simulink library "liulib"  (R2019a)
settings: Solver=ode45  StartTime=0.0  StopTime=10.0  RelTol=1e-3  EnableMultiTasking=on
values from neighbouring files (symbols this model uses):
  ag = NaN(L.ng,1)    [bdet.m]
  D = meqp()    [fbtp.m]
  dr2FA = dr2Fs(1:nA,1)    [asxycs.m]
  drzFA = drzFs(1:nA,1)    [asxycs.m]
  dz = dzxs(is)    [asxycsJac.m]    (also in bintc.m = (z - zx(kz))/dzx)
  dz2FA = dz2Fs(1:nA,1)    [asxycs.m]
  err = [IaeH            ; IoeH               ; IueH               ; DeH               ; FeH            ; BeH               ; BeH               ; BeH               ; CeH               ; CeH               ; CeH               ; VeH                ; VeH                ; VeH               ]    [fbtopt.m]
  FA = Fs(1:nA,1)    [asxycs.m]    (also in bfhelp.m = [-1                        0        0       ])
  FB = [0                         1        1       ]    [bfhelp.m]
  Fx = meqFx(L,Iy,[Ia;Iu])    [bdet.m]    (also in bfhelp.m = zeros(n+2,3); Fx(2:end-1,2) = FN)
  FX = Fs(nA+1:ns,1)    [asxycs.m]
  IpD = LXs.Ip    [fbtinit.m]
  Iy = LXt.Iy    [bdet.m]    (also in fbtinit.m = meqinitIy(L,LXs.t,IpD,bbs,LXs.capaj))
  L = fbtc(P,G)    [fbt.m]    (also in fbtc.m = meqc(P,G); fbte.m = varargout{1})
  nA = numel(rA)    [asxycs.m]
  niter = L.P.itercs    [asxycs.m]
  Opy = logical(Opy)    [bfct.m]    (also in bfdoublet.m = Opy==1 | Opy==2)
  rA = rs(1:nA,1)    [asxycs.m]    (also in fbtptcv.m = (rA1 + 3*rA2)/4)
  rX = rs(nA+1:ns,1)    [asxycs.m]    (also in fbtptcv.m = rzbro(iX,1); fbtxana.m = r0)
  zA = zs(1:nA,1)    [asxycs.m]    (also in fbtptcv.m = (zA1 + 3*zA2)/4)
  zX = zs(nA+1:ns,1)    [asxycs.m]    (also in fbtptcv.m = rzbro(iX,2); fbtxana.m = 0)
undefined symbols (not defined in the file or in its folder): aminor, aq, aW, Bm, bp, bpli2, Brn, Brrn, Brzn, bt, Bzn, Bzrn, Bzzn, delta, deltal, deltau, dzg, epsilon, Ff, Fn, Ft, Ft0, FW, Ie, Ip, iqQ, iTQ, jtorQ, kappa, lB, li, lp, lX, mu, nX, PpQ, PQ, Q0Q, Q1Q, Q2Q, Q3Q, Q4Q, q95, qmin, raQ, raqmin, rB, rbary, rBt, repmat, rgeom, rIp, rIpD, Row, rq, rS, rst, rYD, TQ, TTpQ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
libraries: $bdroot x53, mkllib x48, simulink x7
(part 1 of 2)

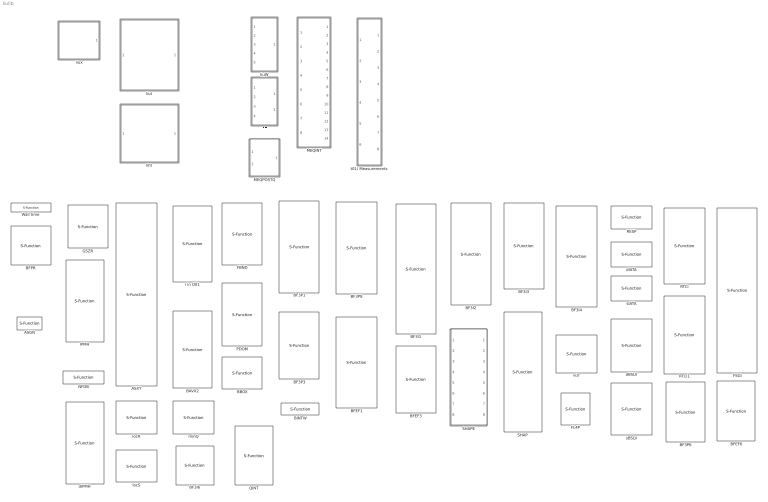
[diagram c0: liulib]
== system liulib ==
  ASGN : S-Function  FunctionName=sasgncsf  Parameters=iu  SFunctionDeploymentMode=off  EnableBusSupport=off  mask{iu=0}
  ASXY : S-Function  FunctionName=sasxycsf  Parameters=rx zx dr dz idr idz Oasx daxm  SFunctionDeploymentMode=off  EnableBusSupport=off  mask{rx=L.G.rx, zx=L.G.zx, dr=L.drx, dz=L.dzx, idr=L.idrx, idz=L.idzx, Oasx=L.Oasx, daxm=L.P.daxm}
      mask prompts: rx "rx [28]"; zx "zx [65]"
      mask help: Axis and Saddle point finder on xy grid
  BAVX2 : S-Function  FunctionName=sbavx2csf  Parameters=a  SFunctionDeploymentMode=off  EnableBusSupport=off  mask{a=0}
      mask prompts: a "alpha"
  BBOX : S-Function  FunctionName=sbboxcsf  Parameters=z r  SFunctionDeploymentMode=off  EnableBusSupport=off  mask{z=L.zy, r=L.ry}
  BF3I1 : S-Function  FunctionName=sbf3i1csf  Parameters=r ir nz nr  SFunctionDeploymentMode=off  EnableBusSupport=off  mask{r=L.ry, ir=L.iry, nz=L.nzy, nr=L.nry}
      mask prompts: r "r inner grid"; ir "ir inner grid"; nz "nzy"; nr "nry"
  BF3I2 : S-Function  FunctionName=sbf3i2csf  SFunctionDeploymentMode=off  EnableBusSupport=off
  BF3I3 : S-Function  FunctionName=sbf3i3csf  Parameters=idsx  SFunctionDeploymentMode=off  EnableBusSupport=off  mask{idsx=L.idsx}
  BF3I4 : S-Function  FunctionName=sbf3i4csf  Parameters=nzy nry  SFunctionDeploymentMode=off  EnableBusSupport=off  mask{nzy=L.nzy, nry=L.nry}
  BF3I6 : S-Function  FunctionName=sbf3i6csf  SFunctionDeploymentMode=off  EnableBusSupport=off
  BF3P1 : S-Function  FunctionName=sbf3p1csf  Parameters=ry iry nzy nry  SFunctionDeploymentMode=off  EnableBusSupport=off  mask{ry=L.ry, iry=L.iry, nzy=L.nzy, nry=L.nry}
      mask prompts: ry "ry inner grid"; iry "iry inner grid"
  BF3P3 : S-Function  FunctionName=sbf3p3csf  Parameters=idsx  SFunctionDeploymentMode=off  EnableBusSupport=off  mask{idsx=L.idsx}
  BF3P6 : S-Function  FunctionName=sbf3p6csf  SFunctionDeploymentMode=off  EnableBusSupport=off
  BF3P8 : S-Function  FunctionName=sbf3p8csf  Parameters=ids iry  SFunctionDeploymentMode=off  EnableBusSupport=off  mask{ids=L.idsx, iry=L.iry}
      mask prompts: ids "r inner grid"; iry "ir inner grid"
  BFEF1 : S-Function  FunctionName=sbfef1csf  Parameters=ry iry nzy nry nP nT  SFunctionDeploymentMode=off  EnableBusSupport=off  mask{ry=L.ry, iry=L.iry, nzy=L.nzy, nry=L.nry, nP=L.P.bfp(1), nT=L.P.bfp(2)}
      mask prompts: ry "ry inner grid"; iry "iry inner grid"
  BFEF3 : S-Function  FunctionName=sbfef3csf  Parameters=ids nP nT  SFunctionDeploymentMode=off  EnableBusSupport=off  mask{ids=L.idsx, nP=L.P.bfp(1), nT=L.P.bfp(2)}
  BFEF6 : S-Function  FunctionName=sbfef6csf  Parameters=nP nT nq  SFunctionDeploymentMode=off  EnableBusSupport=off  mask{nP=L.P.bfp(1), nT=L.P.bfp(2), nq=L.nq}
  BFPR : S-Function  FunctionName=sbfprcsf  SFunctionDeploymentMode=off  EnableBusSupport=off
  BINTW : S-Function  FunctionName=sbintcsf  Parameters=kxW cWx nzx  SFunctionDeploymentMode=off  EnableBusSupport=off  mask{kxW=L.kxW, cWx=L.cWx, nzx=L.nzx}
  FBND : S-Function  FunctionName=sfbndcsf  Parameters=rl zl  SFunctionDeploymentMode=off  EnableBusSupport=off  mask{rl=L.G.rl, zl=L.G.zl}
  FE : Subsystem  Variant=on
  FL4P : S-Function  FunctionName=sfl4pcsf  Parameters=kl cl nz  SFunctionDeploymentMode=off  EnableBusSupport=off  mask{kl=int32(L.kxl-1), cl=L.clx, nz=L.nzx}
      mask prompts: kl "kl 0-based"; cl "cl [4][]"
  FSGI : S-Function  FunctionName=sfsgicsf  Parameters=idoq  SFunctionDeploymentMode=off  EnableBusSupport=off  mask{idoq=1/L.doq}
      mask help: Flux Surface Geometric Integrals
  GSZR : S-Function  FunctionName=sgszrcsf  Parameters=cx cq cr cs ci co  SFunctionDeploymentMode=off  EnableBusSupport=off  mask{cx=L.cx, cq=L.cq, cr=L.cr, cs=L.cs, ci=L.ci, co=L.co}
      mask help: Grad-Shafranov equation on RZ grid
  IPMH : S-Function  FunctionName=sipmhcsf  Parameters=Ahd Aed Ahe Aeh Ahh uAhh nit  SFunctionDeploymentMode=off  EnableBusSupport=off  mask{Ahd=L.Ahd, Aed=L.Aed, Ahe=L.Ahe, Aeh=L.Aeh, Ahh=L.Ahh, uAhh=L.uAhh, nit=L.P.iterh}
      mask prompts: nit "Maximum iteration #"
  MEQINT : Subsystem
  MEQPOSTQ : Subsystem  TreatAsAtomicUnit=on  VariantControl=liuITERQMODEvariant1
  NFDB : S-Function  FunctionName=snfdbcsf  Parameters=nz nr  SFunctionDeploymentMode=off  EnableBusSupport=off  mask{nz=L.nzx, nr=L.nrx}
  PDOM : S-Function  FunctionName=spdomcsf  SFunctionDeploymentMode=off  EnableBusSupport=off
      mask help: Plasma DOmain finder
  QINT : S-Function  FunctionName=sqintcsf  Parameters=rx zx inM  SFunctionDeploymentMode=off  EnableBusSupport=off  mask{rx=L.rx, zx=L.zx, inM=L.inM}
  RESP : S-Function  FunctionName=srespcsf  Parameters=A B nr ng  SFunctionDeploymentMode=off  EnableBusSupport=off  mask{A=L.Wr.*L.Mry, B=L.P.fdz*(L.Wr.*L.Mdzry), nr=L.nr, ng=L.ng}
      mask prompts: A "Mry"; B "Mdzry"
  RTCI : S-Function  FunctionName=srtcicsf  Parameters=c s da nr nz  SFunctionDeploymentMode=off  EnableBusSupport=off  mask{c=L.cdrq, s=L.cdzq, da=L.drx, nr=L.nrx, nz=L.nzx}
      mask prompts: c "cos(theta)*dr"; s "sin(theta)*dz"; da "delta a max"
      mask help: Real-Time Contour Integration
  RTCI1 : S-Function  FunctionName=srtci1csf  SFunctionDeploymentMode=off  EnableBusSupport=off
  SHAP : S-Function  FunctionName=sshapcsf  Parameters=npq noq  SFunctionDeploymentMode=off  EnableBusSupport=off  mask(Computes shape parameters from rq,zq contours){npq=L.npq, noq=L.noq}
      mask help: See shapmex.c, shap.c
  SHAPE : Subsystem  mask(meqshape){npq=L.npq, noq=L.noq}
      mask help: Calculates LCFS shape information. See meqshape.m for details
  Wall time : S-Function  FunctionName=swclkcsf  Parameters=f  SFunctionDeploymentMode=off  EnableBusSupport=off  mask{f=1e6}
      mask prompts: f "Factor (e.g. 1000 for ms)"
  dBSLV : S-Function  FunctionName=dbslvcsf  Parameters=niter  SFunctionDeploymentMode=off  EnableBusSupport=off  mask{niter=L.P.iters}
  dIATA : S-Function  FunctionName=diatacsf  SFunctionDeploymentMode=off  EnableBusSupport=off
  dIPMH : S-Function  FunctionName=dipmhcsf  Parameters=Ahd Aed Ahe Aeh Ahh uAhh nit  SFunctionDeploymentMode=off  EnableBusSupport=off  mask{Ahd=0, Aed=0, Ahe=0, Aeh=0, Ahh=0, uAhh=0, nit=0}
      mask prompts: nit "Maximum iteration #"
  l in OX1 : S-Function  FunctionName=sbavxcsf  Parameters=a  SFunctionDeploymentMode=off  EnableBusSupport=off  mask{a=0}
      mask prompts: a "alpha"
  liht : Subsystem  TreatAsAtomicUnit=on
  liuW : Subsystem  TreatAsAtomicUnit=on
  liut : Subsystem  TreatAsAtomicUnit=on
  liux : Subsystem
  locR : S-Function  FunctionName=slocRcsf  Parameters=nR naR  SFunctionDeploymentMode=off  EnableBusSupport=off  mask{nR=numel(L.P.iqR), naR=1}
  locS : S-Function  FunctionName=slocScsf  SFunctionDeploymentMode=off  EnableBusSupport=off
  minQ : S-Function  FunctionName=sminQcsf  Parameters=nmin  SFunctionDeploymentMode=off  EnableBusSupport=off  mask{nmin=1}
  sBSLV : S-Function  FunctionName=sbslvcsf  Parameters=niter  SFunctionDeploymentMode=off  EnableBusSupport=off  mask{niter=L.P.iters}
  sIATA : S-Function  FunctionName=siatacsf  SFunctionDeploymentMode=off  EnableBusSupport=off
  t01/ Measurements : Subsystem
  vizr : S-Function  FunctionName=svizrcsf  Parameters=ry iry dr dz nr nz  SFunctionDeploymentMode=off  EnableBusSupport=off  mask{ry=L.ry, iry=L.iry, dr=L.drx, dz=L.dzx, nr=L.nrx, nz=L.nzx}
      mask prompts: ry "r inner grid"; iry "ir inner grid"

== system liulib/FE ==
  Yd : Inport
  Ie : Inport  Port=2
  Ip : Inport  Port=3
  sIp : Inport  Port=4
  FE ipm : Subsystem  VariantControl=liuHFCTMODEvariant2
  FE ipm double : Subsystem  VariantControl=liuHFCTMODEvariant3
  FE lsq : Subsystem  VariantControl=liuHFCTMODEvariant1
  Jh : Outport
  Je : Outport  Port=2

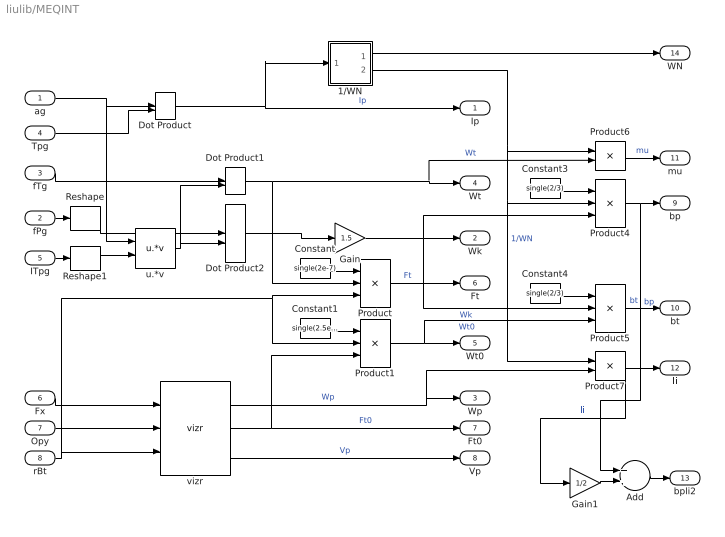
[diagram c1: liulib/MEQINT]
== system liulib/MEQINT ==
  ag : Inport
  fPg : Inport  Port=2
  fTg : Inport  Port=3
  Tpg : Inport  Port=4
  ITpg : Inport  Port=5
  Fx : Inport  Port=6
  Opy : Inport  Port=7
  rBt : Inport  Port=8
  1/WN : Subsystem
  Add : Sum
  Constant : Constant  Value=single(2e-7)  OutDataTypeStr=single
  Constant1 : Constant  Value=single(2.5e6)  OutDataTypeStr=single
  Constant3 : Constant  Value=single(2/3)  OutDataTypeStr=single
  Constant4 : Constant  Value=single(2/3)  OutDataTypeStr=single
  Dot Product : DotProduct
  Dot Product1 : DotProduct
  Dot Product2 : DotProduct
  Gain : Gain  Gain=1.5
  Gain1 : Gain  Gain=1/2
  Product : Product  Inputs=**/
  Product1 : Product  Inputs=3
  Product4 : Product  Inputs=3
  Product5 : Product  Inputs=**/
  Product6 : Product
  Product7 : Product
  Reshape : Reshape
  Reshape1 : Reshape
  u.*v : mkllib/u.*v
  vizr : $bdroot/vizr  ry=L.ry  iry=L.iry  dr=L.drx  dz=L.dzx  nr=L.nrx  nz=L.nzx
  Ip : Outport
  Wk : Outport  Port=2
  Wp : Outport  Port=3
  Wt : Outport  Port=4
  Wt0 : Outport  Port=5
  Ft : Outport  Port=6
  Ft0 : Outport  Port=7
  Vp : Outport  Port=8
  bp : Outport  Port=9
  bt : Outport  Port=10
  mu : Outport  Port=11
  li : Outport  Port=12
  bpli2 : Outport  Port=13
  WN : Outport  Port=14
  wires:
  1/WN/1(WN) -> WN/1
  Gain1/1 -> Add/2
  Add/1 -> bpli2/1
  vizr/3 -> Vp/1  "Vp"
  Fx/1 -> vizr/1
  rBt/1 -> Product1/2, Product/3, vizr/3
  ag/1 -> u.*v/1, Dot Product/1
  Tpg/1 -> Dot Product/2
  u.*v/1 -> Dot Product1/2, Dot Product2/2
  Dot Product/1 -> 1/WN/1(Ip), Ip/1  "Ip"
  Dot Product2/1 -> Gain/1
  vizr/1 -> Product7/2, Wp/1  "Wp"
  Dot Product1/1 -> Product/2, Product6/2, Wt/1  "Wt"
  fTg/1 -> Dot Product1/1
  vizr/2 -> Ft0/1, Product1/3  "Ft0"
  Constant/1 -> Product/1
  Product/1 -> Ft/1  "Ft"
  Constant1/1 -> Product1/1
  Product1/1 -> Product5/3, Wt0/1  "Wt0"
  Constant3/1 -> Product4/1
  Product4/1 -> bp/1, Add/1  "bp"
  Product5/1 -> bt/1  "bt"
  Constant4/1 -> Product5/1
  Product6/1 -> mu/1  "mu"
  Product7/1 -> li/1, Gain1/1  "li"
  Gain/1 -> Product5/2, Product4/3, Wk/1  "Wk"
  1/WN/2(1/WN) -> Product6/1, Product7/1, Product4/2  "1/WN"
  fPg/1 -> Reshape/1
  ITpg/1 -> Reshape1/1
  Reshape/1 -> Dot Product2/1
  Reshape1/1 -> u.*v/2
  Opy/1 -> vizr/2

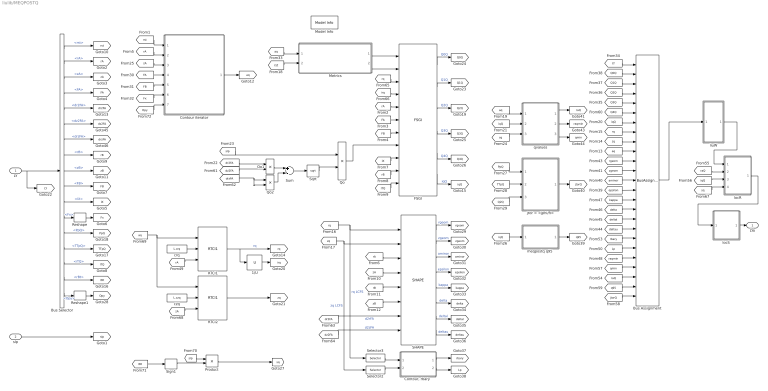
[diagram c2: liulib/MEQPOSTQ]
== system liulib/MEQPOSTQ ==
  LY : Inport
  sIp : Inport  Port=2
  1/U : mkllib/1//U
  Bus Assignment : BusAssignment  AssignedSignals=Q0Q,Q1Q,Q2Q,Q3Q,Q4Q,iqQ,rq,zq,aq,rgeom,zgeom,aminor,epsilon,kappa,delta,deltal,deltau,rbary,lp,raqmin,qmin,raQ,q95,jtorQ
  Bus Selector : BusSelector  OutputSignals=rst,rA,zA,FA,dr2FA,dz2FA,drzFA,rB,zB,FB,lX,Fx,PpQ,TTpQ,iTQ,rBt,Opy
  Contour iterator : Subsystem
  "Contour, rbary " : Subsystem
  FSGI : $bdroot/FSGI  idoq=1/L.doq
  Metrics : Subsystem
  Model Info : simulink/Model-Wide Utilities/Model Info  Frame=on  DisplayStringWithTags=|  HorizontalTextAlignment=Center  LeftAlignmentValue=0.5
      | Model Info
      | %<Creator>
      | %<ModifiedBy>
      | %<ModifiedDate>
      | %<ModifiedComment>
      | %<ModelVersion>
  Product : Product
  Qo : Product  Inputs=**
  Qo1 : Product  Inputs=**
  Qo2 : Product  Inputs=**
  RTCI1 : $bdroot/RTCI1  SFunctionModules=''
  RTCI2 : $bdroot/RTCI1  SFunctionModules=''
  Reshape : Reshape  OutputDimensions=L.nzx*L.nrx
  Reshape1 : Reshape  OutputDimensions=L.nzy*L.nry
  SHAPE : $bdroot/SHAPE  npq=L.npq  noq=L.noq
  Selector2 : Selector  NumberOfDimensions=2  InputPortWidth=3  IndexOptions=Select all,Index vector (dialog)  Indices=[1 3],L.npq  OutputSizes=1,1
  Selector3 : Selector  NumberOfDimensions=2  InputPortWidth=3  IndexOptions=Select all,Index vector (dialog)  Indices=[1 3],L.npq  OutputSizes=1,1
  Sign1 : Signum
  Sqrt : Sqrt
  Sum : Sum  Inputs=+-
  crq : Constant  Value=L.crq  OutDataTypeStr=single
  czq : Constant  Value=L.czq  OutDataTypeStr=single
  jtor = <jphi/R> : Subsystem
  liuW : Subsystem  Variant=on  VariantControl=Variant1
  locR : Subsystem  Variant=on  VariantControl=Variant1
  locS : Subsystem  Variant=on  VariantControl=Variant1
  "meqpostq q95 " : Subsystem
  qvalues : Subsystem
  LYo : Outport
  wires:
  "Contour, rbary "/1(rbary) -> [rbary]
  "Contour, rbary "/2(Lp) -> [Lp]
  qvalues/2(raqmin) -> [raqmin]
  qvalues/3(qmin) -> [qmin]
  [iTQ] -> FSGI/11
  FSGI/1 -> [Q0Q]  "Q0Q"
  Bus Selector/5 -> [dr2FA]  "<dr2FA>"
  SHAPE/3 -> [aminor]  "aminor"
  Bus Selector/4 -> [FA]  "<FA>"
  SHAPE/1 -> [rgeom]  "rgeom"
  SHAPE/8 -> [deltau]  "deltau"
  [rq] -> SHAPE/1, Selector3/1  "rq LCFS"
  [sIp] -> Qo/1
  [iqQ] -> qvalues/2(iqQ)
  Selector2/1 -> "Contour, rbary "/2(zq)
  Bus Selector/2 -> [rA]  "<rA>"
  SHAPE/6 -> [delta]  "delta"
  [rB] -> FSGI/10
  Bus Selector/3 -> [zA]  "<zA>"
  FSGI/4 -> [Q3Q]  "Q3Q"
  Sum/1 -> Sqrt/1
  [zq] -> SHAPE/2, Selector2/1  "zq LCFS"
  [FB] -> FSGI/7
  Metrics/1(da^2/pdp = M1q) -> FSGI/1
  FSGI/6 -> [iqQ]  "iqQ"
  Sqrt/1 -> Qo/2
  [dz2FA] -> SHAPE/8  "d2zFA"
  [sq] -> qvalues/3(sq)
  [aq] -> qvalues/1(aq)
  [dr2FA] -> Qo1/1
  [rst] -> Metrics/2(rst)
  [rB] -> SHAPE/5
  FSGI/2 -> [Q1Q]  "Q1Q"
  [zA] -> SHAPE/4
  Qo1/1 -> Sum/1
  Selector3/1 -> "Contour, rbary "/1(rq)
  SHAPE/4 -> [epsilon]  "epsilon"
  SHAPE/2 -> [zgeom]  "zgeom"
  SHAPE/7 -> [deltal]  "deltal"
  [drzFA] -> Qo2/2, Qo2/1
  [rA] -> SHAPE/3
  [rA] -> FSGI/5
  Qo/1 -> FSGI/8
  [FA] -> FSGI/6
  Qo2/1 -> Sum/2
  Metrics/2(((da^2/2do)^2+a^2)/(da^2/pdp) = M2q) -> FSGI/2
  [zB] -> SHAPE/6
  [lX] -> FSGI/9
  [dr2FA] -> SHAPE/7  "d2rFA"
  SHAPE/5 -> [kappa]  "kappa"
  [dz2FA] -> Qo1/2
  sIp/1 -> [sIp]
  FSGI/3 -> [Q2Q]  "Q2Q"
  FSGI/5 -> [Q4Q]  "Q4Q"
  Bus Selector/1 -> [rst]  "<rst>"
  [iqQ] -> "meqpostq q95 "/1(iqQ)
  "meqpostq q95 "/1(q95) -> [q95]
  [PpQ] -> jtor = <jphi/R>/1(PpQ)
  [TTpQ] -> jtor = <jphi/R>/2(TTpQ)
  [Q2Q] -> jtor = <jphi/R>/3(Q2Q)
  jtor = <jphi/R>/1(jtorQ) -> [jtorQ]
  qvalues/1(raQ) -> [raQ]
  [zA] -> Contour iterator/3(zA)
  [FB] -> Contour iterator/5(FB)
  [rst] -> Contour iterator/1(rst)
  [rA] -> Contour iterator/2(rA)
  [FA] -> Contour iterator/4(FA)
  [Fx] -> Contour iterator/6(Fx)
  Contour iterator/1(aq) -> [aq]
  [aq] -> Metrics/1(aq)
  LY/1 -> [LY], Bus Selector/1
  [jtorQ] -> Bus Assignment/25
  [q95] -> Bus Assignment/24
  [Lp] -> Bus Assignment/20
  [rbary] -> Bus Assignment/19
  [deltau] -> Bus Assignment/18
  [deltal] -> Bus Assignment/17
  [delta] -> Bus Assignment/16
  [kappa] -> Bus Assignment/15
  [epsilon] -> Bus Assignment/14
  [aminor] -> Bus Assignment/13
  [zgeom] -> Bus Assignment/12
  [rgeom] -> Bus Assignment/11
  [aq] -> Bus Assignment/10
  [zq] -> Bus Assignment/9
  [rq] -> Bus Assignment/8
  [iqQ] -> Bus Assignment/7
  [Q4Q] -> Bus Assignment/6
  [Q3Q] -> Bus Assignment/5
  [Q2Q] -> Bus Assignment/4
  [Q1Q] -> Bus Assignment/3
  [Q0Q] -> Bus Assignment/2
  [LY] -> Bus Assignment/1
  Bus Selector/6 -> [dz2FA]  "<dz2FA>"
  Bus Selector/7 -> [drzFA]  "<drzFA>"
  Bus Selector/8 -> [rB]  "<rB>"
  Bus Selector/9 -> [zB]  "<zB>"
  Bus Selector/10 -> [FB]  "<FB>"
  Bus Selector/11 -> [lX]  "<lX>"
  Bus Selector/13 -> [PpQ]  "<PpQ>"
  Bus Selector/14 -> [TTpQ]  "<TTpQ>"
  Bus Selector/15 -> [iTQ]  "<iTQ>"
  Reshape/1 -> [Fx]
  Bus Selector/12 -> Reshape/1  "<Fx>"
  [irq] -> FSGI/4
  [rq] -> FSGI/3
  locS/1(" LYo") -> LYo/1
  Bus Assignment/1 -> liuW/1(LY)
  [raQ] -> locR/2("raQ ")
  [iqQ] -> locR/3("qQ ")
  [sq] -> locR/4(sq)
  liuW/1(LYo) -> locR/1(LY)
  locR/1(" LYo") -> locS/1("LY ")
  [raqmin] -> Bus Assignment/21
  [qmin] -> Bus Assignment/22
  [raQ] -> Bus Assignment/23
  RTCI1/1 -> [rq], 1/U/1  "rq"
  crq/1 -> RTCI1/2
  czq/1 -> RTCI2/2
  [zA] -> RTCI2/3
  [aq] -> RTCI2/1, RTCI1/1
  [rA] -> RTCI1/3
  1/U/1 -> [irq]
  RTCI2/1 -> [zq]
  Sign1/1 -> Product/2
  [sIp] -> Product/1
  Product/1 -> [sq]
  Bus Selector/16 -> [rBt]  "<rBt>"
  [rBt] -> Sign1/1
  [Opy] -> Contour iterator/7(Opy)
  Bus Selector/17 -> Reshape1/1  "<Opy>"
  Reshape1/1 -> [Opy]

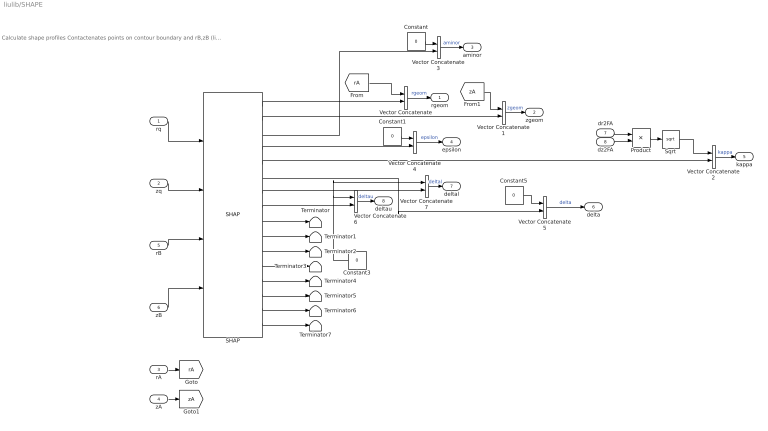
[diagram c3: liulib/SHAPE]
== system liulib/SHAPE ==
  note: Calculate shape profiles Contactenates points on contour boundary and rB,zB (limiter/divertor point) see also meqshape.m
  rq : Inport  OutDataTypeStr=single
  zq : Inport  Port=2  OutDataTypeStr=single
  rA : Inport  Port=3  OutDataTypeStr=single
  zA : Inport  Port=4  OutDataTypeStr=single
  rB : Inport  Port=5  OutDataTypeStr=single
  zB : Inport  Port=6  OutDataTypeStr=single
  dr2FA : Inport  Port=7
  dz2FA : Inport  Port=8
  Constant{,1,3,5} (4 alike) : Constant  Value=0  OutDataTypeStr=single
  Product : Product  Inputs=*/
  SHAP : $bdroot/SHAP  npq=L.npq  noq=L.noq
  Sqrt : Sqrt
  Terminator{,1..7} (8 alike) : Terminator
  Vector Concatenate{,1..7} (8 alike) : Concatenate
  rgeom : Outport
  zgeom : Outport  Port=2
  aminor : Outport  Port=3
  epsilon : Outport  Port=4
  kappa : Outport  Port=5
  delta : Outport  Port=6
  deltal : Outport  Port=7
  deltau : Outport  Port=8
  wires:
  SHAP/6 -> Vector Concatenate5/2
  SHAP/4 -> Vector Concatenate4/2
  rq/1 -> SHAP/1
  zq/1 -> SHAP/2
  zB/1 -> SHAP/4
  rB/1 -> SHAP/3
  SHAP/1 -> Vector Concatenate/2
  SHAP/3 -> Vector Concatenate3/2
  SHAP/5 -> Vector Concatenate2/2
  SHAP/7 -> Vector Concatenate7/2
  SHAP/9 -> Terminator/1
  SHAP/8 -> Vector Concatenate6/2
  SHAP/10 -> Terminator1/1
  SHAP/11 -> Terminator2/1
  SHAP/12 -> Terminator3/1
  SHAP/13 -> Terminator4/1
  SHAP/14 -> Terminator5/1
  SHAP/15 -> Terminator6/1
  SHAP/16 -> Terminator7/1
  Vector Concatenate/1 -> rgeom/1  "rgeom"
  rA/1 -> [rA]
  [rA] -> Vector Concatenate/1
  zA/1 -> [zA]
  [zA] -> Vector Concatenate1/1
  SHAP/2 -> Vector Concatenate1/2
  Vector Concatenate1/1 -> zgeom/1  "zgeom"
  Vector Concatenate2/1 -> kappa/1  "kappa"
  Vector Concatenate3/1 -> aminor/1  "aminor"
  Vector Concatenate4/1 -> epsilon/1  "epsilon"
  Constant/1 -> Vector Concatenate3/1
  Constant1/1 -> Vector Concatenate4/1
  Vector Concatenate5/1 -> delta/1  "delta"
  Vector Concatenate6/1 -> deltau/1  "deltau"
  Constant3/1 -> Vector Concatenate7/1, Vector Concatenate6/1
  Vector Concatenate7/1 -> deltal/1  "deltal"
  Constant5/1 -> Vector Concatenate5/1
  Product/1 -> Sqrt/1
  Sqrt/1 -> Vector Concatenate2/1
  dz2FA/1 -> Product/2
  dr2FA/1 -> Product/1

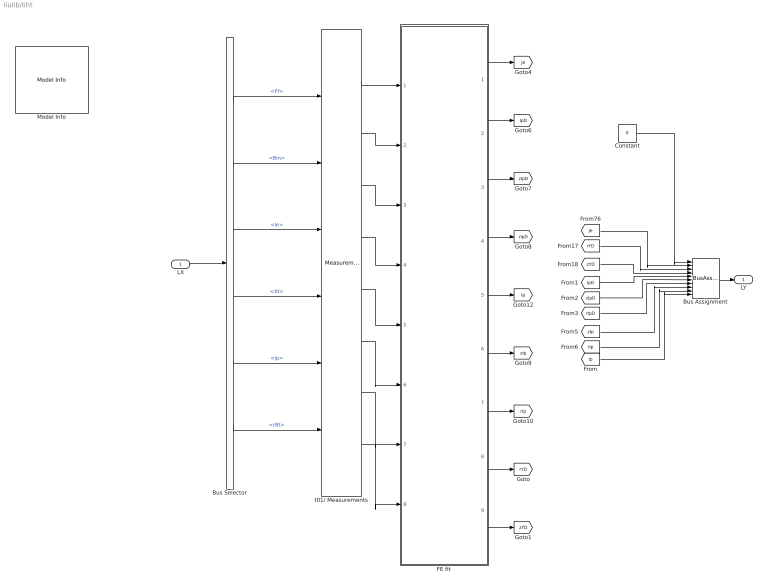
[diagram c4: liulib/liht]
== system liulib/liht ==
  LX : Inport
  Bus Assignment : BusAssignment  AssignedSignals=Ie,rYD,zYD,IpD,zIpD,rIpD,zIp,rIp,Ip
  Bus Selector : BusSelector  OutputSignals=Ff,Bm,Ie,Xt,Ip,rBt
  Constant : Constant  Value=0  OutDataTypeStr=Bus: LYbus
  FE fit : Subsystem
  Model Info : simulink/Model-Wide Utilities/Model Info  Frame=on  DisplayStringWithTags=|  HorizontalTextAlignment=Center  LeftAlignmentValue=0.5
      | Model Info
      | %<Creator>
      | %<ModifiedBy>
      | %<ModifiedDate>
      | %<ModifiedComment>
      | %<ModelVersion>
  t01/ Measurements : $bdroot/t01// Measurements  SystemSampleTime=-1  Latency=0  AutoFrameSizeCalculation=off
  LY : Outport
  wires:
  FE fit/6(Out7) -> [zIp]
  FE fit/7(Out8) -> [rIp]
  FE fit/5(Out9) -> [Ip]
  FE fit/8(Out5) -> [rYD]
  [Ip] -> Bus Assignment/10
  [rIp] -> Bus Assignment/9
  [zIp] -> Bus Assignment/8
  Bus Assignment/1 -> LY/1
  Bus Selector/6 -> t01/ Measurements/6  "<rBt>"
  Bus Selector/4 -> t01/ Measurements/4  "<Xt>"
  t01/ Measurements/4 -> FE fit/4(Ie)
  Bus Selector/3 -> t01/ Measurements/3  "<Ie>"
  Bus Selector/5 -> t01/ Measurements/5  "<Ip>"
  LX/1 -> Bus Selector/1
  t01/ Measurements/8 -> FE fit/8(sIp)
  t01/ Measurements/7 -> FE fit/7(FN)
  t01/ Measurements/6 -> FE fit/6(rBt)
  t01/ Measurements/5 -> FE fit/5(Ip)
  t01/ Measurements/3 -> FE fit/3(Yi)
  t01/ Measurements/2 -> FE fit/2(Yd)
  Bus Selector/1 -> t01/ Measurements/1  "<Ff>"
  Bus Selector/2 -> t01/ Measurements/2  "<Bm>"
  t01/ Measurements/1 -> FE fit/1(Yr)
  FE fit/1(Out4) -> [Je]
  FE fit/9(Out6) -> [zYD]
  FE fit/2(Out1) -> [IpD]
  FE fit/3(Out2) -> [zIpD]
  FE fit/4(Out3) -> [rIpD]
  Constant/1 -> Bus Assignment/1
  [Je] -> Bus Assignment/2
  [IpD] -> Bus Assignment/5
  [zIpD] -> Bus Assignment/6
  [rIpD] -> Bus Assignment/7
  [rYD] -> Bus Assignment/3
  [zYD] -> Bus Assignment/4

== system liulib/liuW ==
  zaW : Inport
  rst : Inport  Port=2
  FW : Inport  Port=3
  Fx : Inport  Port=4
  Opy : Inport  Port=5
  BINTW : $bdroot/BINTW  kxW=L.kxW  cWx=L.cWx  nzx=L.nzx
  Constant : Constant  Value=int8(0)
  IC = 1 : UnitDelay  InitialCondition=1  SampleTime=-1  HasFrameUpgradeWarning=on
  RTCI : $bdroot/RTCI  c=L.cdrW  s=L.cdzW  da=L.drx  nr=L.nrx  nz=L.nzx
  Reshape1 : Reshape
  Reshape2 : Reshape
  "aq " : Switch  Criteria=u2 ~= 0
  dan : Terminator
  rx1 : Constant  Value=L.erW  OutDataTypeStr=single
  rx2 : Constant  Value=L.ezW  OutDataTypeStr=single
  rx3 : Constant  Value=zeros(L.G.nW,L.P.nFW)  VectorParams1D=off  OutDataTypeStr=single
  aW : Outport
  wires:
  Reshape2/1 -> RTCI/6
  Reshape1/1 -> BINTW/1, RTCI/4
  rst/1 -> IC = 1/1
  zaW/1 -> "aq "/3
  FW/1 -> RTCI/5
  "aq "/1 -> RTCI/1
  RTCI/2 -> dan/1
  rx1/1 -> RTCI/2
  rx2/1 -> RTCI/3
  Fx/1 -> Reshape1/1
  rx3/1 -> "aq "/1
  RTCI/1 -> aW/1  "aW"
  BINTW/1 -> RTCI/7
  Constant/1 -> RTCI/8
  Opy/1 -> Reshape2/1
  IC = 1/1 -> "aq "/2

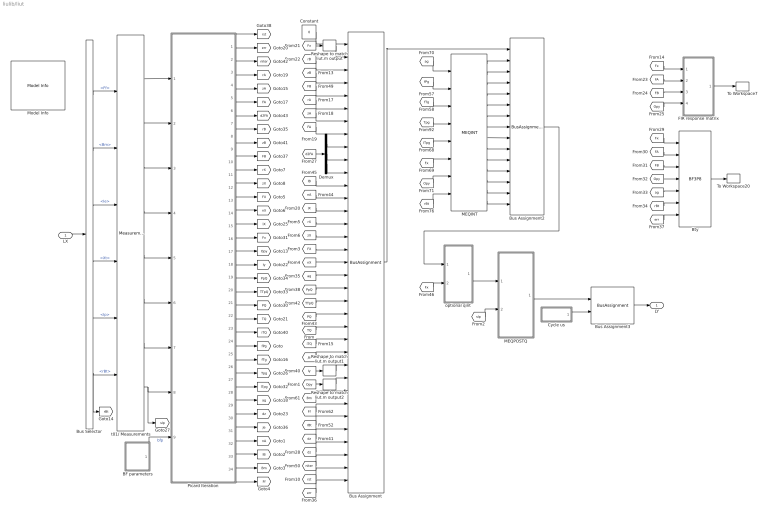
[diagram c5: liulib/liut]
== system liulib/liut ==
  LX : Inport
  BF parameters : Subsystem  Variant=on  VariantControl=Variant1
  Bty : $bdroot/BF3P8  Commented=on  ids=L.idsx  iry=L.iry
  Bus Assignment : BusAssignment  AssignedSignals=Fx,rB,zB,FB,rA,zA,FA,dr2FA,dz2FA,drzFA,lB,nA,lX,rX,zX,FX,nX,ag,PpQ,TTpQ,PQ,TQ,iTQ,Ie,Iy,Opy,Bm,Ff,rBt,dz,dzg,niter,rst,err
  Bus Assignment2 : BusAssignment  AssignedSignals=Ip,Wk,Wp,Wt,Wt0,Ft,Ft0,Vp,bp,bt,mu,li,bpli2,WN
  Bus Assignment3 : BusAssignment  AssignedSignals=cycle
  Bus Selector : BusSelector  OutputSignals=Ff,Bm,Ie,Xt,Ip,rBt
  Constant : Constant  Value=0  OutDataTypeStr=Bus: LYbus
  Cycle us : Subsystem
  Demux : Demux  Outputs=3
  FIR response matrix : Subsystem  Commented=on
  MEQINT : $bdroot/MEQINT  SystemSampleTime=-1
  MEQPOSTQ : Subsystem  Variant=on  VariantControl=Variant1
  Model Info : simulink/Model-Wide Utilities/Model Info  Frame=on  DisplayStringWithTags=|  HorizontalTextAlignment=Center  LeftAlignmentValue=0.5
      | Model Info
      | %<Creator>
      | %<ModifiedBy>
      | %<ModifiedDate>
      | %<ModifiedComment>
      | %<ModelVersion>
  Picard Iteration : Subsystem
  Reshape to match liut.m output : Reshape  OutputDimensionality=Customize  OutputDimensions=[L.nzx,L.nrx]
  Reshape to match liut.m output1 : Reshape  OutputDimensionality=Customize  OutputDimensions=[L.nzy,L.nry]
  Reshape to match liut.m output2 : Reshape  OutputDimensionality=Customize  OutputDimensions=[L.nzy,L.nry]
  To Workspace20 : ToWorkspace  VariableName=Bty  SampleTime=-1
  To Workspace7 : ToWorkspace  VariableName=Tdg  SampleTime=-1
  optional qint : Subsystem  Variant=on  VariantControl=Variant1
  t01/ Measurements : $bdroot/t01// Measurements  SystemSampleTime=-1
  LY : Outport
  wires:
  [zX] -> Bus Assignment/16
  [rX] -> Bus Assignment/15
  Picard Iteration/12(Out34) -> [zX]
  Picard Iteration/11(Out33) -> [rX]
  [nX] -> Bus Assignment/18
  Picard Iteration/14(Out32) -> [nX]
  [FX] -> Bus Assignment/17
  Bus Assignment2/1 -> optional qint/1("LY ")
  [Fx] -> optional qint/2(Fx)
  Picard Iteration/34(Out30) -> [Ff]
  Picard Iteration/33(Out29) -> [Bm]
  MEQINT/14 -> Bus Assignment2/15
  [iTQ] -> Bus Assignment/24
  Reshape to match liut.m output1/1 -> Bus Assignment/26
  [Iy] -> Reshape to match liut.m output1/1
  [Je] -> Bus Assignment/25
  Bus Selector/6 -> t01/ Measurements/6, [rBt]  "<rBt>"
  Bus Selector/4 -> t01/ Measurements/4  "<Xt>"
  [Opy] -> FIR response matrix/4(Opy)
  [FA] -> Bty/2
  [FA] -> FIR response matrix/2(FA)
  FIR response matrix/1(Tdg) -> To Workspace7/1
  [Opy] -> Bty/4
  [rBt] -> Bty/6
  Bty/1 -> To Workspace20/1
  [Fx] -> FIR response matrix/1(Fx)
  [ag] -> Bty/5
  [FB] -> FIR response matrix/3(FB)
  [Fx] -> Bty/1
  [FB] -> Bty/3
  [err] -> Bty/7
  Bus Assignment3/1 -> LY/1
  Cycle us/1(Out1) -> Bus Assignment3/2
  Reshape to match liut.m output/1 -> Bus Assignment/2
  MEQINT/13 -> Bus Assignment2/14
  Bus Assignment/1 -> Bus Assignment2/1
  [TQ] -> Bus Assignment/23
  [PQ] -> Bus Assignment/22
  [TTpQ] -> Bus Assignment/21
  [PpQ] -> Bus Assignment/20
  [lX] -> Bus Assignment/14
  [ag] -> Bus Assignment/19
  [nA] -> Bus Assignment/13
  [lB] -> Bus Assignment/12
  Picard Iteration/32(Out28) -> [lB]
  Picard Iteration/31(Out27) -> [nA]
  [Fx] -> Reshape to match liut.m output/1
  [rB] -> Bus Assignment/3
  [zB] -> Bus Assignment/4
  [FB] -> Bus Assignment/5
  [d2FA] -> Demux/1
  Demux/2 -> Bus Assignment/10
  Demux/3 -> Bus Assignment/11
  Demux/1 -> Bus Assignment/9
  [FA] -> Bus Assignment/8
  [zA] -> Bus Assignment/7
  [rA] -> Bus Assignment/6
  Picard Iteration/23(Out18) -> [iTQ]
  Picard Iteration/19(Out25) -> [PpQ]
  Picard Iteration/29(Out24) -> [dz]
  Picard Iteration/18(Out15) -> [Iy]
  Picard Iteration/5(Out6) -> [zA]
  Picard Iteration/30(Out4) -> [Je]
  Picard Iteration/20(Out26) -> [TTpQ]
  Picard Iteration/10(Out11) -> [FB]
  Picard Iteration/27(Out22) -> [ITpg]
  Picard Iteration/22(Out17) -> [TQ]
  Picard Iteration/17(Out14) -> [Opy]
  Picard Iteration/15(Out12) -> [lX]
  Picard Iteration/1(Out1) -> [rst]
  Picard Iteration/3(Out3) -> [niter]
  Picard Iteration/16(Out13) -> [Fx]
  Picard Iteration/28(Out23) -> [ag]
  Picard Iteration/26(Out21) -> [Tpg]
  Picard Iteration/25(Out20) -> [fTg]
  Picard Iteration/7(Out8) -> [d2FA]
  Picard Iteration/21(Out16) -> [PQ]
  Picard Iteration/2(Out2) -> [err]
  Picard Iteration/4(Out5) -> [rA]
  Picard Iteration/9(Out10) -> [zB]
  Picard Iteration/24(Out19) -> [fPg]
  Picard Iteration/6(Out7) -> [FA]
  Picard Iteration/8(Out9) -> [rB]
  Constant/1 -> Bus Assignment/1
  MEQINT/10 -> Bus Assignment2/11
  MEQINT/11 -> Bus Assignment2/12
  MEQINT/8 -> Bus Assignment2/9
  [ITpg] -> MEQINT/5
  MEQINT/4 -> Bus Assignment2/5
  [Tpg] -> MEQINT/4
  MEQINT/2 -> Bus Assignment2/3
  [Fx] -> MEQINT/6
  MEQINT/1 -> Bus Assignment2/2
  MEQINT/12 -> Bus Assignment2/13
  MEQINT/7 -> Bus Assignment2/8
  MEQINT/9 -> Bus Assignment2/10
  [rBt] -> MEQINT/8
  MEQINT/6 -> Bus Assignment2/7
  [fPg] -> MEQINT/2
  MEQINT/3 -> Bus Assignment2/4
  [fTg] -> MEQINT/3
  [Opy] -> MEQINT/7
  [ag] -> MEQINT/1
  MEQINT/5 -> Bus Assignment2/6
  t01/ Measurements/4 -> Picard Iteration/4(Ie)
  Bus Selector/3 -> t01/ Measurements/3  "<Ie>"
  Bus Selector/5 -> t01/ Measurements/5  "<Ip>"
  LX/1 -> Bus Selector/1
  BF parameters/1(" bfp") -> Picard Iteration/9(bfp)  "bfp"
  t01/ Measurements/8 -> Picard Iteration/8(sIp), [sIp]
  t01/ Measurements/7 -> Picard Iteration/7(FN)
  t01/ Measurements/6 -> Picard Iteration/6(rBt)
  t01/ Measurements/3 -> Picard Iteration/3(Yi)
  t01/ Measurements/2 -> Picard Iteration/2(Yd)
  Bus Selector/1 -> t01/ Measurements/1  "<Ff>"
  Bus Selector/2 -> t01/ Measurements/2  "<Bm>"
  t01/ Measurements/1 -> Picard Iteration/1(Yr)
  optional qint/1(" LYo") -> MEQPOSTQ/1("LY ")
  [sIp] -> MEQPOSTQ/2("sIp ")
  MEQPOSTQ/1(" LYo") -> Bus Assignment3/1
  [Bm] -> Bus Assignment/28
  [rBt] -> Bus Assignment/30
  [Ff] -> Bus Assignment/29
  [dz] -> Bus Assignment/31
  [dz] -> Bus Assignment/32
  [niter] -> Bus Assignment/33
  [rst] -> Bus Assignment/34
  [err] -> Bus Assignment/35
  [Opy] -> Reshape to match liut.m output2/1
  Reshape to match liut.m output2/1 -> Bus Assignment/27
  t01/ Measurements/5 -> Picard Iteration/5(Ip)
  Picard Iteration/13(Out31) -> [FX]

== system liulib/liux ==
  Bm1 : FromWorkspace  VariableName=struct('time',[],'signals',struct('values',single(LX.Bm')))  SampleTime=L.dt  Interpolate=off  OutputAfterFinalValue=Holding final value
  Bus Assignment : BusAssignment  AssignedSignals=Ff,Bm,Ie,Xt,Ip,rBt
  Constant : Constant  Value=0  OutDataTypeStr=Bus: LXbus
  Ff1 : FromWorkspace  VariableName=struct('time',[],'signals',struct('values',single(LX.Ff')))  SampleTime=L.dt  Interpolate=off  OutputAfterFinalValue=Holding final value
  Ft1 : FromWorkspace  VariableName=struct('time',[],'signals',struct('values',single(LX.Xt')))  SampleTime=L.dt  Interpolate=off  OutputAfterFinalValue=Holding final value
  Ft2 : FromWorkspace  VariableName=struct('time',[],'signals',struct('values',single(LX.Ip')))  SampleTime=L.dt  Interpolate=off  OutputAfterFinalValue=Holding final value
  Ia1 : FromWorkspace  VariableName=struct('time',[],'signals',struct('values',single(LX.Ie')))  SampleTime=L.dt  Interpolate=off  OutputAfterFinalValue=Holding final value
  RBt1 : FromWorkspace  VariableName=struct('time',[],'signals',struct('values',single(LX.rBt')))  SampleTime=L.dt  Interpolate=off  OutputAfterFinalValue=Holding final value
  LX : Outport  OutDataTypeStr=Bus: LXbus
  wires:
  Constant/1 -> Bus Assignment/1
  Bus Assignment/1 -> LX/1
  Ft2/1 -> Bus Assignment/6  "Ip"
  RBt1/1 -> Bus Assignment/7  "rBt"
  Ft1/1 -> Bus Assignment/5  "Xt"
  Ia1/1 -> Bus Assignment/4  "Ia"
  Bm1/1 -> Bus Assignment/3  "Bm"
  Ff1/1 -> Bus Assignment/2  "Ff"

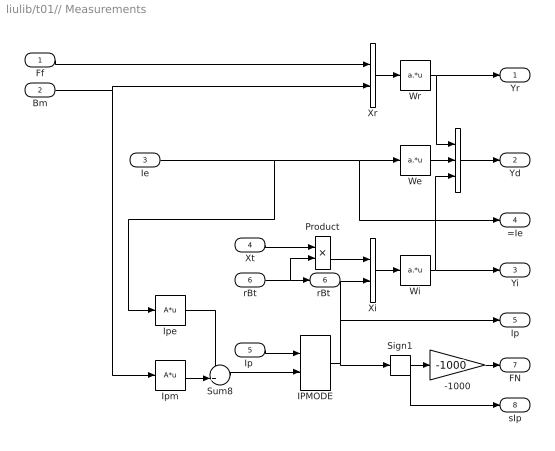
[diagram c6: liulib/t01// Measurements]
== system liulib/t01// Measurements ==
  Ff : Inport
  Bm : Inport  Port=2
  Ie : Inport  Port=3
  Xt : Inport  Port=4
  "Ip " : Inport  Port=5
  rBt : Inport  Port=6
  " " : Concatenate  NumInputs=3
  -1000 : Gain  Gain=-1000
  IPMODE : VariantSource
  Ipe : mkllib/A*u  A=single([L.Ipa L.Ipu])
  Ipm : mkllib/A*u  A=single(L.G.Ipm)
  Product : Product
  Sign1 : Signum
  Sum8 : Sum  Inputs=++|
  We : mkllib/a.*u  a=single(L.We)
  Wi : mkllib/a.*u  a=single(L.Wi)
  Wr : mkllib/a.*u  a=single(L.Wr)
  Xi : Concatenate
  Xr : Concatenate
  Yr : Outport
  Yd : Outport  Port=2
  Yi : Outport  Port=3
  =Ie : Outport  Port=4
  Ip : Outport  Port=5
  "rBt " : Outport  Port=6
  FN : Outport  Port=7
  sIp : Outport  Port=8
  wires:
  " "/1 -> Yd/1
  We/1 -> " "/2
  Wi/1 -> Yi/1, " "/3
  Wr/1 -> Yr/1, " "/1
  Xi/1 -> Wi/1
  Xr/1 -> Wr/1
  Product/1 -> Xi/1
  Xt/1 -> Product/1
  rBt/1 -> Product/2, "rBt "/1
  IPMODE/1 -> Ip/1, Xi/2, Sign1/1
  Sign1/1 -> sIp/1, -1000/1
  -1000/1 -> FN/1
  Ipm/1 -> Sum8/2
  Ipe/1 -> Sum8/1
  "Ip "/1 -> IPMODE/1
  Sum8/1 -> IPMODE/2
  Ff/1 -> Xr/1
  Ie/1 -> Ipe/1, We/1, =Ie/1
  Bm/1 -> Xr/2, Ipm/1

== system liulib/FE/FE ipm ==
  Yd : Inport
  Ie : Inport  Port=2
  Ip : Inport  Port=3
  sIp : Inport  Port=4
  1/nh : Constant  Value=repmat(single(1/L.nh),L.nh,1)  OutDataTypeStr=single
  Divide : Product  Inputs=**
  Divide1 : Product  Inputs=***
  IPMH : $bdroot/IPMH  Ahd=L.Ahd  Aed=L.Aed  Ahe=L.Ahe  Aeh=L.Aeh  Ahh=L.Ahh  uAhh=L.uAhh  nit=L.P.iterh
  Terminator1 : Terminator
  tolh/nh : Constant  Value=single(L.P.tolh/L.nh)  OutDataTypeStr=single
  Jh : Outport
  Je : Outport  Port=2
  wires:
  Ip/1 -> Divide1/2, Divide/1
  Yd/1 -> IPMH/1
  Ie/1 -> IPMH/2
  sIp/1 -> IPMH/4, Divide1/1
  IPMH/2 -> Jh/1
  IPMH/1 -> Je/1
  IPMH/3 -> Terminator1/1
  1/nh/1 -> Divide/2
  Divide1/1 -> IPMH/5
  Divide/1 -> IPMH/3
  tolh/nh/1 -> Divide1/3

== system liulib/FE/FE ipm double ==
  Yd : Inport
  Ie : Inport  Port=2
  Ip : Inport  Port=3
  sIp : Inport  Port=4
  1/nh : Constant  Value=repmat(1/L.nh,L.nh,1)  OutDataTypeStr=double
  Data Type Conversion{,1..3} (4 alike) : DataTypeConversion  OutDataTypeStr=double
  Data Type Conversion4 : DataTypeConversion  OutDataTypeStr=single
  Data Type Conversion5 : DataTypeConversion  OutDataTypeStr=single
  Divide : Product  Inputs=**
  Divide1 : Product  Inputs=***
  Terminator1 : Terminator
  dIPMH : $bdroot/dIPMH  Ahd=double(L.Ahd)  Aed=double(L.Aed)  Ahe=double(L.Ahe)  Aeh=double(L.Aeh)  Ahh=double(L.Ahh)  uAhh=double(L.uAhh)  nit=L.P.iterh
  tolh/nh : Constant  Value=L.P.tolh/L.nh  OutDataTypeStr=double
  Jh : Outport
  Je : Outport  Port=2
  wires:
  Ie/1 -> Data Type Conversion1/1
  1/nh/1 -> Divide/2
  Divide/1 -> dIPMH/3
  sIp/1 -> Data Type Conversion3/1
  dIPMH/1 -> Data Type Conversion4/1
  dIPMH/3 -> Terminator1/1
  tolh/nh/1 -> Divide1/3
  Divide1/1 -> dIPMH/5
  dIPMH/2 -> Data Type Conversion5/1
  Ip/1 -> Data Type Conversion2/1
  Yd/1 -> Data Type Conversion/1
  Data Type Conversion/1 -> dIPMH/1
  Data Type Conversion1/1 -> dIPMH/2
  Data Type Conversion2/1 -> Divide1/2, Divide/1
  Data Type Conversion3/1 -> dIPMH/4, Divide1/1
  Data Type Conversion4/1 -> Je/1
  Data Type Conversion5/1 -> Jh/1

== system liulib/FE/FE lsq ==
  Yd : Inport
  Ie : Inport  Port=2
  Ip : Inport  Port=3
  sIp : Inport  Port=4
  Aed : mkllib/A*u  A=L.Aed
  Ahd : mkllib/A*u  A=L.Ahd
  Terminator : Terminator
  Terminator1 : Terminator
  Terminator2 : Terminator
  Jh : Outport
  Je : Outport  Port=2
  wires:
  Ahd/1 -> Jh/1
  Yd/1 -> Aed/1, Ahd/1
  Aed/1 -> Je/1
  Ie/1 -> Terminator/1
  Ip/1 -> Terminator1/1
  sIp/1 -> Terminator2/1

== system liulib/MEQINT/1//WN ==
  note: WN=(\mu_0 I_p^2)/4
  Ip : Inport
  1./u : mkllib/1.//u
  Constant1 : Constant  Value=0  OutDataTypeStr=single
  Constant2 : Constant  Value=single(1/(1e-7*pi*L.P.r0))  OutDataTypeStr=single
  Product1 : Product  Inputs=*/
  Product2 : Product
  Switch : Switch  Criteria=u2 ~= 0
  WN : Outport
  1/WN : Outport  Port=2
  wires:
  1./u/1 -> Switch/1
  Product1/1 -> WN/1, 1./u/1
  Ip/1 -> Switch/2, Product2/2, Product2/1
  Constant2/1 -> Product1/2
  Product2/1 -> Product1/1
  Switch/1 -> 1/WN/1
  Constant1/1 -> Switch/3

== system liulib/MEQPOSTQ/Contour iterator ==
  rst : Inport
  rA : Inport  Port=2
  zA : Inport  Port=3
  FA : Inport  Port=4
  FB : Inport  Port=5
  Fx : Inport  Port=6
  Opy : Inport  Port=7
  Flux contours : Subsystem  TreatAsAtomicUnit=on
  For Iterator : ForIterator  IterationLimit=L.P.iterq  ShowIterationPort=off
  Unit Delay : UnitDelay  SampleTime=-1  HasFrameUpgradeWarning=on
  aq : Outport
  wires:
  rst/1 -> Flux contours/2(rst)
  rA/1 -> Flux contours/3(rA)
  zA/1 -> Flux contours/4(zA)
  Unit Delay/1 -> Flux contours/1(zaq)
  Fx/1 -> Flux contours/7(Fx)
  FA/1 -> Flux contours/5(FA)
  FB/1 -> Flux contours/6(FB)
  Flux contours/1(aq) -> Unit Delay/1, aq/1
  Opy/1 -> Flux contours/8(Opy)

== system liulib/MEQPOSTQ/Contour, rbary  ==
  rq : Inport
  zq : Inport  Port=2
  Divide : Product  Inputs=*/
  Dot Product : DotProduct
  Gain : Gain  Gain=1/2
  Product : Product
  Product1 : Product
  Selector4 : Selector  NumberOfDimensions=2  IndexOptions=Index vector (dialog),Select all  Indices=[2:L.noq,1],1  OutputSizes=1,1
  Selector5 : Selector  NumberOfDimensions=2  IndexOptions=Index vector (dialog),Select all  Indices=[2:L.noq,1],1  OutputSizes=1,1
  Sqrt1 : Sqrt
  Subtract : Sum  Inputs=+-
  Subtract1 : Sum  Inputs=+-
  Subtract2 : Sum
  Subtract3 : Sum
  Sum of Elements : Sum  Inputs=+
  rbary : Outport
  Lp : Outport  Port=2
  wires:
  Divide/1 -> rbary/1  "rbary"
  zq/1 -> Selector5/1, Subtract1/2
  rq/1 -> Selector4/1, Subtract/2, Subtract3/2
  Subtract/1 -> Product/1, Product/2
  Subtract2/1 -> Sqrt1/1
  Sum of Elements/1 -> Lp/1, Divide/2  "Lp"
  Subtract3/1 -> Gain/1
  Gain/1 -> Dot Product/1  "R(q) trapezoidal"
  Selector4/1 -> Subtract/1, Subtract3/1
  Product/1 -> Subtract2/1
  Selector5/1 -> Subtract1/1
  Subtract1/1 -> Product1/1, Product1/2
  Product1/1 -> Subtract2/2
  Dot Product/1 -> Divide/1
  Sqrt1/1 -> Dot Product/2, Sum of Elements/1  "dq"

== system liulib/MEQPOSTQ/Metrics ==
  aq : Inport
  rst : Inport  Port=2
  *M1q : mkllib/U*A  A=L.M1q
  Constant : Constant  Value=zeros(L.noq,L.npq)  OutDataTypeStr=single
  Coq : Product  Inputs=/*
  M2q* : mkllib/A*U  A=L.M2q
  Product : Product
  Product2 : Product  Inputs=/**
  Switch : Switch  Criteria=u2 > Threshold
  Switch1 : Switch  Criteria=u2 > Threshold
  qaq1 : Sum  Inputs=|++
  da^2/pdp = M1q : Outport
  ((da^2/2do)^2+a^2)/(da^2/pdp) = M2q : Outport  Port=2
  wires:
  aq/1 -> Product/1, Product/2
  Product/1 -> *M1q/1, M2q*/1, Product2/1, qaq1/1
  *M1q/1 -> Coq/1, Switch/3
  M2q*/1 -> Product2/2, Product2/3
  Product2/1 -> qaq1/2
  qaq1/1 -> Coq/2
  Coq/1 -> Switch1/3
  Switch/1 -> da^2/pdp = M1q/1
  rst/1 -> Switch1/2, Switch/2
  Constant/1 -> Switch1/1, Switch/1
  Switch1/1 -> ((da^2/2do)^2+a^2)/(da^2/pdp) = M2q/1

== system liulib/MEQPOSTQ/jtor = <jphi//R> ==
  PpQ : Inport
  TTpQ : Inport  Port=2
  Q2Q : Inport  Port=3
  Add : Sum
  Gain : Gain  Gain=single(2*pi*L.P.r0)
  Gain1 : Gain  Gain=single(1/(4e-7*pi))
  Product : Product
  jtorQ : Outport
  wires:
  TTpQ/1 -> Product/1
  PpQ/1 -> Add/1
  Q2Q/1 -> Product/2
  Gain/1 -> jtorQ/1
  Product/1 -> Gain1/1
  Add/1 -> Gain/1
  Gain1/1 -> Add/2

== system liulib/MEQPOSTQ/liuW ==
  LY : Inport
  dummy : Subsystem  VariantControl=liuAWMODEvariant0
  liuW : Subsystem  VariantControl=liuAWMODEvariant1
  LYo : Outport

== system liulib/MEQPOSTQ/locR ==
  LY : Inport
  "raQ " : Inport  Port=2
  "qQ " : Inport  Port=3
  sq : Inport  Port=4
  dummy : Subsystem  VariantControl=liuLOCRMODEvariant0
  locR : Subsystem  VariantControl=liuLOCRMODEvariant1
  " LYo" : Outport

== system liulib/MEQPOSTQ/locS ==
  "LY " : Inport
  dummy : Subsystem  VariantControl=liuLOCSMODEvariant0
  locS : Subsystem  VariantControl=liuLOCSMODEvariant1
  " LYo" : Outport

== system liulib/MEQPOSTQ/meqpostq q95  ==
  iqQ : Inport
  1./u : mkllib/1.//u
  Gain : Gain  Gain=L.c95  Multiplication=Matrix(K*u) (u vector)
  Selector4 : Selector  IndexOptions=Index vector (dialog)  Indices=L.i95  OutputSizes=1
  q95 : Outport
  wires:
  Gain/1 -> 1./u/1
  iqQ/1 -> Selector4/1
  Selector4/1 -> Gain/1
  1./u/1 -> q95/1

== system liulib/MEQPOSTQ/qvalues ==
  aq : Inport
  iqQ : Inport  Port=2
  sq : Inport  Port=3
  1/U : mkllib/1//U
  Constant4 : Constant  Value=L.raN  OutDataTypeStr=single
  Gain : Gain  Gain=-1
  Normalized Radius : Subsystem
  minQ : $bdroot/minQ  nmin=1
  raQ : Outport
  raqmin : Outport  Port=2
  qmin : Outport  Port=3
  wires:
  1/U/1 -> qmin/1
  Constant4/1 -> minQ/4
  minQ/1 -> raqmin/1
  minQ/2 -> 1/U/1
  sq/1 -> Gain/1
  Normalized Radius/1(raQ) -> minQ/1, raQ/1
  aq/1 -> Normalized Radius/1(aq)
  iqQ/1 -> minQ/2
  Gain/1 -> minQ/3

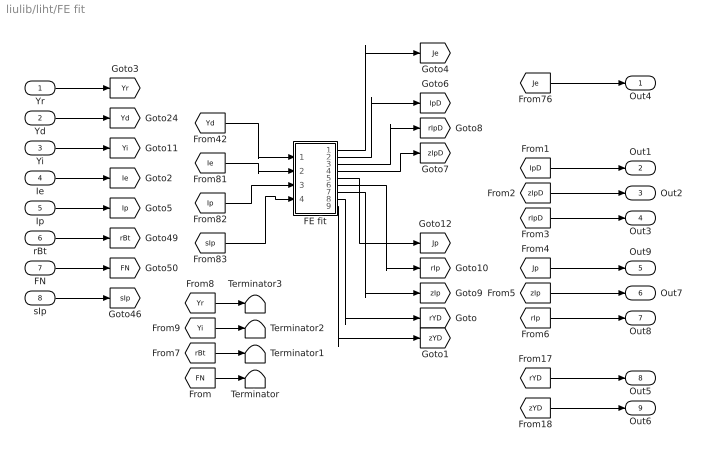
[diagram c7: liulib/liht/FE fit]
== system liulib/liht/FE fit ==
  Yr : Inport
  Yd : Inport  Port=2
  Yi : Inport  Port=3
  Ie : Inport  Port=4
  Ip : Inport  Port=5
  rBt : Inport  Port=6
  FN : Inport  Port=7
  sIp : Inport  Port=8
  FE fit : Subsystem
  Terminator{,1..3} (4 alike) : Terminator
  Out4 : Outport
  Out1 : Outport  Port=2
  Out2 : Outport  Port=3
  Out3 : Outport  Port=4
  Out9 : Outport  Port=5
  Out7 : Outport  Port=6
  Out8 : Outport  Port=7
  Out5 : Outport  Port=8
  Out6 : Outport  Port=9
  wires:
  FE fit/9(zYD) -> [zYD]
  FE fit/8(rYD) -> [rYD]
  rBt/1 -> [rBt]
  FN/1 -> [FN]
  sIp/1 -> [sIp]
  Yr/1 -> [Yr]
  Yi/1 -> [Yi]
  Ip/1 -> [Ip]
  Yd/1 -> [Yd]
  Ie/1 -> [Ie]
  [zYD] -> Out6/1
  [rYD] -> Out5/1
  [Je] -> Out4/1
  [Yd] -> FE fit/1(Yd)
  [Ie] -> FE fit/2(Ie)
  [Ip] -> FE fit/3(Ip_in)
  [sIp] -> FE fit/4(sIp)
  FE fit/1(Je) -> [Je]
  FE fit/5(Ip) -> [Jp]
  FE fit/7(zIp) -> [zIp]
  FE fit/6(rIp) -> [rIp]
  FE fit/3(rIpD) -> [rIpD]
  FE fit/4(zIpD) -> [zIpD]
  FE fit/2(IpD) -> [IpD]
  [IpD] -> Out1/1
  [zIpD] -> Out2/1
  [rIpD] -> Out3/1
  [zIp] -> Out7/1
  [rIp] -> Out8/1
  [Jp] -> Out9/1
  [FN] -> Terminator/1
  [rBt] -> Terminator1/1
  [Yi] -> Terminator2/1
  [Yr] -> Terminator3/1

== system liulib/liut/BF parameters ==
  BF3I : Subsystem  VariantControl=liuBFCTMODEvariant2
  BF3P : Subsystem  VariantControl=liuBFCTMODEvariant1
  BFEF : Subsystem  VariantControl=liuBFCTMODEvariant3
  " bfp" : Outport

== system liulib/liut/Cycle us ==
  Data Type Conversion : DataTypeConversion
  Memory : Memory  InheritSampleTime=on
  Sum : Sum  Inputs=|+-
  Wall time : $bdroot/Wall time  f=1000000
  Out1 : Outport  OutDataTypeStr=single
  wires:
  Data Type Conversion/1 -> Out1/1
  Memory/1 -> Sum/2, Wall time/1
  Sum/1 -> Data Type Conversion/1
  Wall time/1 -> Memory/1, Sum/1

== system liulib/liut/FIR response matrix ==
  Fx : Inport
  FA : Inport  Port=2
  FB : Inport  Port=3
  Opy : Inport  Port=4
  BF3I4 : $bdroot/BF3I4  nzy=L.nzy  nry=L.nry
  Constant : Constant  Value=ones(21,3)  VectorParams1D=off  OutDataTypeStr=single
  Constant1 : Constant  Value=0:9  OutDataTypeStr=uint32
  Constant2 : Constant  Value=[ones(10,1) zeros(10,1)]  OutDataTypeStr=single
  Terminator : Terminator
  Tdg : Outport
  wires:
  FB/1 -> BF3I4/3
  BF3I4/1 -> Tdg/1
  Constant/1 -> BF3I4/5
  Constant1/1 -> BF3I4/6
  FA/1 -> BF3I4/2
  Constant2/1 -> BF3I4/7
  Opy/1 -> BF3I4/4
  Fx/1 -> BF3I4/1
  BF3I4/2 -> Terminator/1

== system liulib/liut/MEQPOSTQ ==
  "LY " : Inport
  "sIp " : Inport  Port=2
  Direct pass : Subsystem  VariantControl=liuITERQMODEvariant0
  MEQPOSTQ : $bdroot/MEQPOSTQ  SystemSampleTime=-1  VariantControl=liuITERQMODEvariant1
  " LYo" : Outport

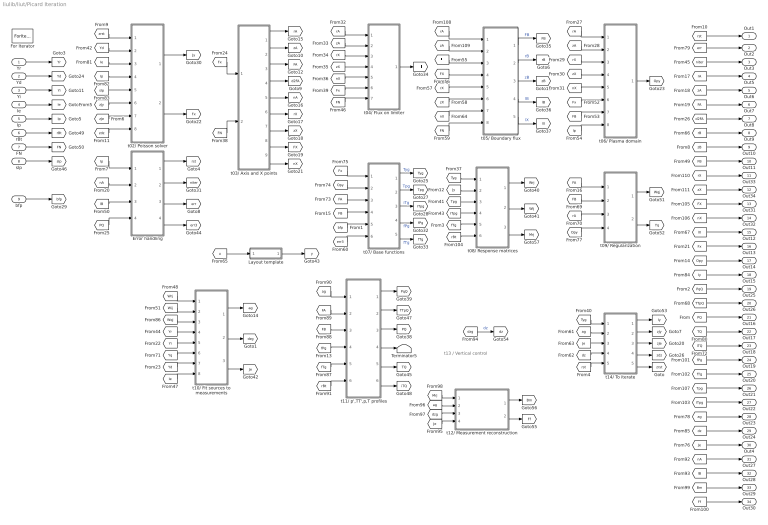
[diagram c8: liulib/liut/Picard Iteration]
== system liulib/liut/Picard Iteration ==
  note: t13 / Vertical control
  Yr : Inport
  Yd : Inport  Port=2
  Yi : Inport  Port=3
  Ie : Inport  Port=4
  Ip : Inport  Port=5
  rBt : Inport  Port=6
  FN : Inport  Port=7
  sIp : Inport  Port=8
  bfp : Inport  Port=9
  Error handling : Subsystem
  For Iterator : ForIterator  IterationLimit=L.P.itert  ShowIterationPort=off
  Layout template : Subsystem  Commented=on
  Terminator5 : Terminator
  t02/ Poisson solver : Subsystem
  t03/ Axis and X points : Subsystem  TreatAsAtomicUnit=on
  t04/ Flux on limiter : Subsystem
  t05/ Boundary flux : Subsystem
  t06/ Plasma domain : Subsystem
  t07/ Base functions : Subsystem  Variant=on
  t08/ Response matrices : Subsystem
  t09/ Regularization : Subsystem  TreatAsAtomicUnit=on
  t10/ Fit sources to measurements : Subsystem  Variant=on  VariantControl=Variant1
  t11/ p',TT',p,T profiles : Subsystem  VariantControl=Variant1
  t12/ Measurement reconstruction : Subsystem
  t14/ To iterate : Subsystem
  Out1 : Outport
  Out2 : Outport  Port=2
  Out3 : Outport  Port=3
  Out5 : Outport  Port=4
  Out6 : Outport  Port=5
  Out7 : Outport  Port=6
  Out8 : Outport  Port=7
  Out9 : Outport  Port=8
  Out10 : Outport  Port=9
  Out11 : Outport  Port=10
  Out33 : Outport  Port=11
  Out34 : Outport  Port=12
  Out31 : Outport  Port=13
  Out32 : Outport  Port=14
  Out12 : Outport  Port=15
  Out13 : Outport  Port=16
  Out14 : Outport  Port=17
  Out15 : Outport  Port=18
  Out25 : Outport  Port=19
  Out26 : Outport  Port=20
  Out16 : Outport  Port=21
  Out17 : Outport  Port=22
  Out18 : Outport  Port=23
  Out19 : Outport  Port=24
  Out20 : Outport  Port=25
  Out21 : Outport  Port=26
  Out22 : Outport  Port=27
  Out23 : Outport  Port=28
  Out24 : Outport  Port=29
  Out4 : Outport  Port=30
  Out27 : Outport  Port=31
  Out28 : Outport  Port=32
  Out29 : Outport  Port=33
  Out30 : Outport  Port=34
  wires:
  t03/ Axis and X points/9(nX) -> [nX]
  t03/ Axis and X points/8(FX) -> [FX]
  t03/ Axis and X points/7(zX) -> [zX]
  t03/ Axis and X points/6(rX) -> [rX]
  t03/ Axis and X points/5(nA) -> [nA]
  t03/ Axis and X points/4(d2FA) -> [d2FA]
  t03/ Axis and X points/3(FA) -> [FA]
  t03/ Axis and X points/2(zA) -> [zA]
  t03/ Axis and X points/1(rA) -> [rA]
  [FN] -> t03/ Axis and X points/2(FN)
  [Fx] -> t03/ Axis and X points/1(Fx)
  [zX] -> Out34/1
  [rX] -> Out33/1
  [nX] -> Out32/1
  [Bm] -> Out29/1
  [Ff] -> Out30/1
  [Je] -> t12/ Measurement reconstruction/4(Ie)
  t08/ Response matrices/3(Mrj) -> [Mrj]
  [dzg] -> t12/ Measurement reconstruction/3(dzg)
  [ag] -> t12/ Measurement reconstruction/2(ag)
  [Mrj] -> t12/ Measurement reconstruction/1(Mrj)
  t12/ Measurement reconstruction/2(Ff) -> [Ff]
  t12/ Measurement reconstruction/1(Bm) -> [Bm]
  [dzg] -> [dz]  "dz"
  [lB] -> Out28/1
  [nA] -> Out27/1
  t14/ To iterate/1(Iy) -> [Iy]
  [TTpQ] -> Out26/1
  [PqQ] -> Out25/1
  t14/ To iterate/5(zrst) -> [zrst]
  t14/ To iterate/4(zdz) -> [zdz]
  t14/ To iterate/3(zJe) -> [zJe]
  t14/ To iterate/2(zJy) -> [zJy]
  [dz] -> t14/ To iterate/4(dz)
  [Je] -> t14/ To iterate/3(Je)
  [Tyg] -> t14/ To iterate/1(Tyg)
  [ag] -> t14/ To iterate/2(ag)
  [rst] -> t14/ To iterate/5(rst)
  [fPg] -> t11/ p',TT',p,T profiles/4(fPg)
  [ag] -> t11/ p',TT',p,T profiles/1(ag)
  [FA] -> t11/ p',TT',p,T profiles/2(FA)
  [ITpg] -> Out22/1
  rBt/1 -> [rBt]
  FN/1 -> [FN]
  [zB] -> Out10/1
  Error handling/2(niter) -> [niter]
  Error handling/1(rst) -> [rst]
  t08/ Response matrices/1(Wrj) -> [Wrj]
  [Fx] -> t07/ Base functions/1(Fx)
  [Opy] -> t07/ Base functions/2(Opy)
  [FA] -> t07/ Base functions/3(FA)
  t02/ Poisson solver/1(Jy) -> [Jy]
  [zdz] -> t02/ Poisson solver/8(zdz)
  t02/ Poisson solver/2(Fx) -> [Fx]
  [dz] -> Out24/1
  [niter] -> Out3/1
  [lB] -> Error handling/3(lB)
  Error handling/3(err) -> [err]
  [Fx] -> t06/ Plasma domain/6(Fx)
  [FB] -> t06/ Plasma domain/7(FB)
  [Ip] -> t06/ Plasma domain/8(Ip)
  [TQ] -> Out17/1
  [Ie] -> t02/ Poisson solver/3(Ie)
  [Ip] -> t02/ Poisson solver/4(Ip)
  [rBt] -> t11/ p',TT',p,T profiles/6(rBt)
  [err] -> Out2/1
  [ag] -> Out23/1
  [d2FA] -> Out8/1
  [FA] -> Out7/1
  [FB] -> t07/ Base functions/4(FB)
  [err3] -> t07/ Base functions/6(err)
  t07/ Base functions/1(Tyg) -> [Tyg]  "Tyg"
  [bfp] -> t07/ Base functions/5(bfp)
  t07/ Base functions/4(fPg) -> [fPg]  "fPg"
  t07/ Base functions/5(fTg) -> [fTg]  "fTg"
  sIp/1 -> [sIp]
  [sIp] -> t02/ Poisson solver/5(sIp)
  [rst] -> Out1/1
  [Jy] -> t08/ Response matrices/2(Jy)
  t06/ Plasma domain/1(Opy) -> [Opy]
  [Tyg] -> t08/ Response matrices/1(Tyg)
  [Tpg] -> t08/ Response matrices/3(Tpg)
  t11/ p',TT',p,T profiles/1(PpQ) -> [PqQ]
  t11/ p',TT',p,T profiles/2(TTpQ) -> [TTpQ]
  t11/ p',TT',p,T profiles/4(hqTQ) -> Terminator5/1
  [fTg] -> t08/ Response matrices/5(fTg)
  t08/ Response matrices/2(Wij) -> [Wij]
  [zA] -> t06/ Plasma domain/2(zA)
  [zX] -> t06/ Plasma domain/4(zX)
  [nX] -> t06/ Plasma domain/5(nX)
  t11/ p',TT',p,T profiles/5(TQ) -> [TQ]
  t11/ p',TT',p,T profiles/6(iTQ) -> [iTQ]
  [iTQ] -> Out18/1
  [zJy] -> t02/ Poisson solver/6(zJy)
  [Yd] -> t02/ Poisson solver/2(Yd)
  [zJe] -> t02/ Poisson solver/7(zJe)
  Yr/1 -> [Yr]
  Yi/1 -> [Yi]
  Ip/1 -> [Ip]
  bfp/1 -> [bfp]
  [FN] -> t04/ Flux on limiter/7(FN)
  [Fx] -> t04/ Flux on limiter/6(Fx)
  Yd/1 -> [Yd]
  Ie/1 -> [Ie]
  [zrst] -> t02/ Poisson solver/1(rst)
  [FB] -> t11/ p',TT',p,T profiles/3(FB)
  [fTg] -> t11/ p',TT',p,T profiles/5(fTg)
  [rA] -> t06/ Plasma domain/1(rA)
  [rX] -> t06/ Plasma domain/3(rX)
  [zX] -> t04/ Flux on limiter/4(zX)
  [rX] -> t04/ Flux on limiter/3(rX)
  [nX] -> t04/ Flux on limiter/5(nX)
  [Tpg] -> Out21/1
  [fTg] -> Out20/1
  [fPg] -> Out19/1
  [ITpg] -> t08/ Response matrices/4(ITpg)
  t04/ Flux on limiter/1(Fl) -> [Fl]
  [zA] -> Out6/1
  [rA] -> Out5/1
  [rB] -> Out9/1
  [lX] -> Out12/1
  t11/ p',TT',p,T profiles/3(PQ) -> [PQ]
  [Opy] -> Out14/1
  [FB] -> Out11/1
  [Fx] -> Out13/1
  [Ip] -> Error handling/1(Ip)
  [nA] -> Error handling/2(nA)
  [PQ] -> Error handling/4(PQ)
  [Iy] -> Out15/1
  [PQ] -> Out16/1
  Layout template/1(y) -> [y]
  [u] -> Layout template/1(u)
  [rA] -> t04/ Flux on limiter/1(rA)
  [zA] -> t04/ Flux on limiter/2(zA)
  t07/ Base functions/2(Tpg) -> [Tpg]  "Tpg"
  t07/ Base functions/3(ITpg) -> [ITpg]  "iTg"
  Error handling/4(err3) -> [err3]
  [Wrj] -> t10/ Fit sources to measurements/1(Wrj)
  [Wij] -> t10/ Fit sources to measurements/2(Wij)
  [Yr] -> t10/ Fit sources to measurements/4(Yr)
  [Yi] -> t10/ Fit sources to measurements/5(Yi)
  [Yd] -> t10/ Fit sources to measurements/7(Yd)
  [Ie] -> t10/ Fit sources to measurements/8(Ie)
  t10/ Fit sources to measurements/1(ag) -> [ag]
  t10/ Fit sources to measurements/2(dzg) -> [dzg]
  t10/ Fit sources to measurements/3(Je) -> [Je]
  t09/ Regularization/1(Wqj) -> [Wqj]
  t09/ Regularization/2(Yq) -> [Yq]
  [rA] -> t09/ Regularization/3(rA)
  [Opy] -> t09/ Regularization/4(Opy)
  [FB] -> t09/ Regularization/2(FB)
  [FA] -> t09/ Regularization/1(FA)
  [Yq] -> t10/ Fit sources to measurements/6(Yq)
  [Wqj] -> t10/ Fit sources to measurements/3(Wqj)
  [Je] -> Out4/1
  [rBt] -> t08/ Response matrices/6(rBt)
  [FX] -> Out31/1
  [nX] -> t05/ Boundary flux/7(nX)
  [FX] -> t05/ Boundary flux/4(FX)
  [Fl] -> t05/ Boundary flux/3(Fl)
  [rX] -> t05/ Boundary flux/5(rX)
  [zX] -> t05/ Boundary flux/6(zX)
  [FN] -> t05/ Boundary flux/8(FN)
  t05/ Boundary flux/2(rB) -> [rB]  "rB"
  t05/ Boundary flux/3(zB) -> [zB]  "zB"
  t05/ Boundary flux/4(lB) -> [lB]  "lB"
  t05/ Boundary flux/1(FB) -> [FB]  "FB"
  t05/ Boundary flux/5(lX) -> [lX]  "lX"
  [zA] -> t05/ Boundary flux/2(zA)
  [rA] -> t05/ Boundary flux/1(rA)
